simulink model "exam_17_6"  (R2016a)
settings: Solver=ode15s  StartTime=0.0  StopTime=1  RelTol=1e-3
libraries: powerlib x7

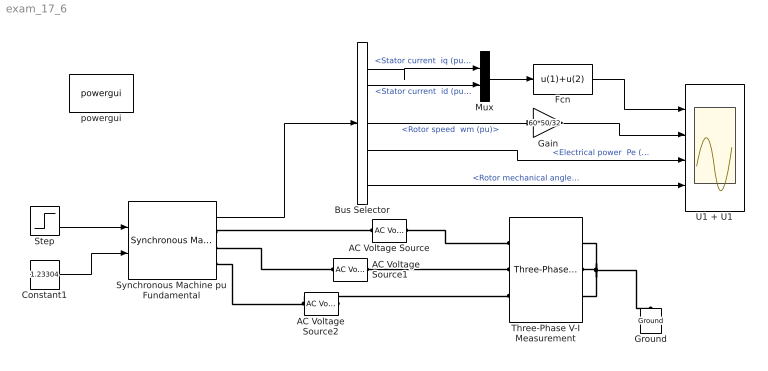
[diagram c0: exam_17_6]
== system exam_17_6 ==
  AC Voltage Source : powerlib/Electrical Sources/AC Voltage Source  Amplitude=10500*1.414/1.732  Phase=0  Frequency=50  SampleTime=0  Measurements=None  BusType=swing  Pref=50e6  Qref=0  Qmin=-inf  Qmax=+inf
  AC Voltage Source1 : powerlib/Electrical Sources/AC Voltage Source  Amplitude=10500*1.414/1.732  Phase=0  Frequency=50  SampleTime=0  Measurements=None  BusType=swing  Pref=50e6  Qref=0  Qmin=-inf  Qmax=+inf
  AC Voltage Source2 : powerlib/Electrical Sources/AC Voltage Source  Amplitude=10500*1.414/1.732  Phase=0  Frequency=50  SampleTime=0  Measurements=None  BusType=swing  Pref=50e6  Qref=0  Qmin=-inf  Qmax=+inf
  Bus Selector : BusSelector  OutputSignals="dq0 components.Stator current  iq (pu),dq0 components.Stator current  id (pu),Mechanical.Rotor speed  wm (pu),Mechanical.Electrical power  Pe (pu),Mechanical.Rotor mechanical angle  theta (deg)"
  Constant1 : Constant  Value=1.23304  VectorParams1D=off
  Fcn : Fcn  Expr=u(1)+u(2)
  Gain : Gain  Gain=60*50/32
  Ground : powerlib/Elements/Ground  LConnTagsString=a
  Mux : Mux  Inputs=2
  Step : Step  Time=0.6  Before=0.8  After=0.6  SampleTime=0.001  VectorParams1D=off  ZeroCross=off
  Synchronous Machine pu Fundamental : powerlib/Machines/Synchronous Machine pu Fundamental  PresetModel=No  MechanicalLoad=Mechanical power Pm  ShowDetailedParameters=on  RotorType=Salient-pole  Units=per unit fundamental parameters  MeasurementBus=off  NominalParameters="[50e6  10.5e3   50]"  Stator="[0.003  0.19837  0.91763  0.21763 ]"  Field="[6.3501e-04  0.16537]"  Dampers2=[0.0652, 0.5134, 0.0287, 0.2553, 7.765e-3, 0.9167 ]  Dampers1="[ 4.6454e-03  3.9203e-02  6.8430e-03  1.4544e-02 ]"  Mechanical="[3.195  0  32]"  PolePairs=20  InitialConditions="[ 0  -71.6365  0.8  0.8  0.8  -0.0279696  -120.02  119.972   1.23304]"  SetSaturation=off  Saturation=[0.6404,0.7127,0.8441,0.9214,0.9956,1.082,1.19,1.316,1.457;0.7,0.7698,0.8872,0.9466,0.9969,1.046,1.1,1.151,1.201]  LoadFlowParameters=[1,0,0,0,0]  TsPowergui=0  TsBlock=-1  IterativeModel=Trapezoidal non iterative  IterativeDiscreteModel=Trapezoidal non iterative  BusType=PV  Pref=0  Qref=0  Qmin=-inf  Qmax=inf  PLF=0  QLF=0
  Three-Phase V-I Measurement : powerlib/Measurements/Three-Phase V-I Measurement  VoltageMeasurement=no  SetLabelV=off  LabelV=Vabc  Vpu=on  VpuLL=off  CurrentMeasurement=no  SetLabelI=off  LabelI=Iabc  Ipu=off  Pbase=100e6  Vbase=500e3  OutputType=Complex  PhasorSimulation=off  PSBequivalent=0
  U1 + U1 : Scope  NumInputPorts=4
  powergui : powerlib/powergui  Priority=1  SimulationMode=Continuous  SolverType=Tustin/Backward Euler (TBE)  SampleTime=50e-6  frequency=60  SPID=off  DisableSnubberDevices=off  DisableRonSwitches=off  DisableVfSwitches=off  SwTol=0  DisplayEquations=off  Interpol=off  ExternalGateDelay=off  methode=off  Ts=10  FunctionMessages=off  echomessages=off  HookPort=off  EnableUseOfTLC=off  x0status=blocks  frequencyindice=50  Pbase=50e6  ErrMax=1e-4  Iterations=50  UnitsV=kV  UnitsW=MW  buscounter=0  RestoreLinks=warning  ResistiveCurrentMeasurement=off  Frange=[0:2:500]  Ylog=off  Xlog=on  ShowGrid=off  save=off  variable=ZData  structure=0  ZoomFFT=off  StartTime=0.0  cycles=1  DisplayStyle=1  fundamental=60  FreqAxis=off  MaxFrequency=1000  frequencyindicesteady=1  RmsSteady=1  display=off
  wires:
  Synchronous Machine pu Fundamental/1 -> Bus Selector/1
  Gain/1 -> U1 + U1/2
  Step/1 -> Synchronous Machine pu Fundamental/1
  Constant1/1 -> Synchronous Machine pu Fundamental/2
  Bus Selector/3 -> Gain/1  "<Rotor speed  wm (pu)>"
  Bus Selector/2 -> Mux/2  "<Stator current  id (pu)>"
  Bus Selector/4 -> U1 + U1/3  "<Electrical power  Pe (pu)>"
  Bus Selector/5 -> U1 + U1/4  "<Rotor mechanical angle  theta (deg)>"
  Bus Selector/1 -> Mux/1  "<Stator current  iq (pu)>"
  Mux/1 -> Fcn/1
  Fcn/1 -> U1 + U1/1
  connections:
  Synchronous Machine pu Fundamental/RConn1 -- AC Voltage Source/RConn1
  AC Voltage Source/LConn1 -- Three-Phase V-I Measurement/LConn1
  Synchronous Machine pu Fundamental/RConn2 -- AC Voltage Source1/RConn1
  AC Voltage Source1/LConn1 -- Three-Phase V-I Measurement/LConn2
  Synchronous Machine pu Fundamental/RConn3 -- AC Voltage Source2/RConn1
  AC Voltage Source2/LConn1 -- Three-Phase V-I Measurement/LConn3
  Three-Phase V-I Measurement/RConn2 -- Three-Phase V-I Measurement/RConn1 -- Three-Phase V-I Measurement/RConn3 -- Ground/LConn1
